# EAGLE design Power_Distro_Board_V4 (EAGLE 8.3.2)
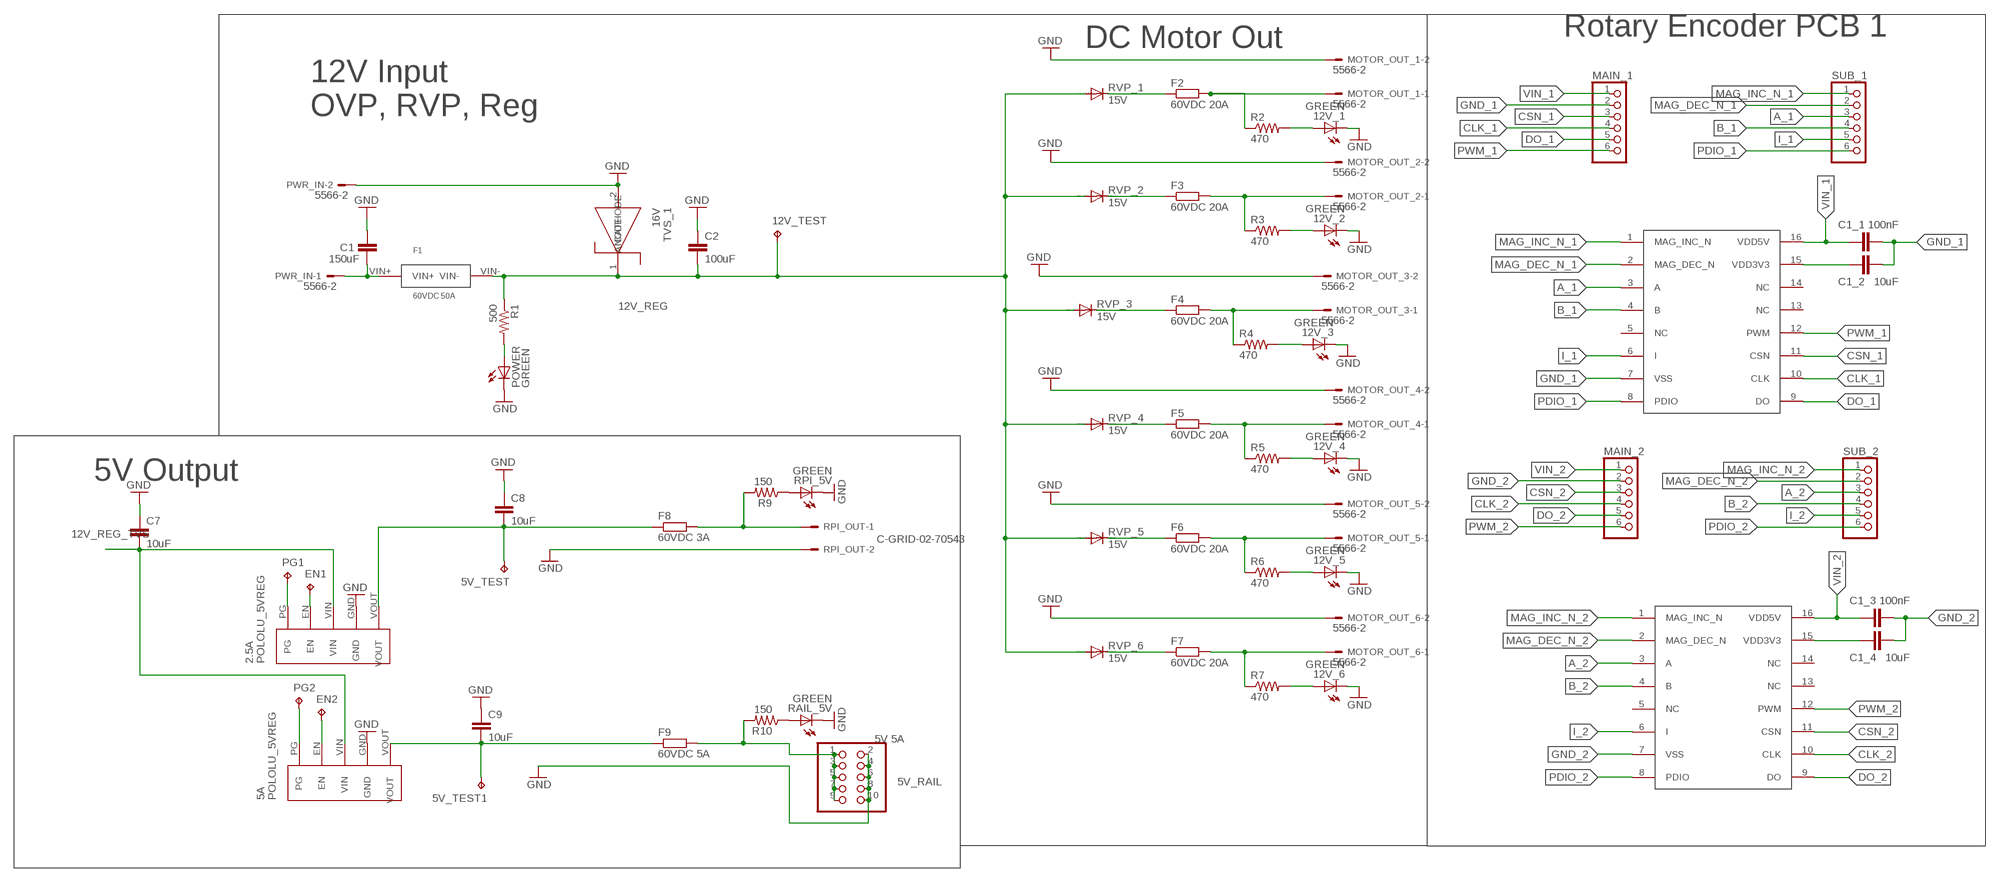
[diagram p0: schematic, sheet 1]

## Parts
2.5A  POLOLU_5VREG  [SIP5]
5A  POLOLU_5VREG  [SIP5]
5V_RAIL  5V 5A  PINHD-2X5  [2X05]
5V_TEST  TPPAD1-13  [P1-13]
5V_TEST1  TPPAD1-13  [P1-13]
12V_1  GREEN  LEDSML1206  [SML1206]
12V_2  GREEN  LEDSML1206  [SML1206]
12V_3  GREEN  LEDSML1206  [SML1206]
12V_4  GREEN  LEDSML1206  [SML1206]
12V_5  GREEN  LEDSML1206  [SML1206]
12V_6  GREEN  LEDSML1206  [SML1206]
12V_TEST  TPPAD1-13  [P1-13]
C1  150uF  C-EUC1206  [C1206]
C1_1  100nF  C-EUC1206  [C1206]
C1_2  10uF  C-EUC1206  [C1206]
C1_3  100nF  C-EUC1206  [C1206]
C1_4  10uF  C-EUC1206  [C1206]
C2  100uF  C-EUC1206  [C1206]
C7  10uF  C-EUC1206  [C1206]
C8  10uF  C-EUC1206  [C1206]
C9  10uF  C-EUC1206  [C1206]
EN1  TPPAD1-13  [P1-13]
EN2  TPPAD1-13  [P1-13]
ENC_1  ENCODER_AS5045B  [SSOP16]
ENC_2  ENCODER_AS5045B  [SSOP16]
F1  60VDC 50A  LITTLEFUSENANO463  [NANO]
F2  60VDC 20A  R-EU_R1206W  [R1206W]
F3  60VDC 20A  R-EU_R1206W  [R1206W]
F4  60VDC 20A  R-EU_R1206W  [R1206W]
F5  60VDC 20A  R-EU_R1206W  [R1206W]
F6  60VDC 20A  R-EU_R1206W  [R1206W]
F7  60VDC 20A  R-EU_R1206W  [R1206W]
F8  60VDC 3A  R-EU_R1206W  [R1206W]
F9  60VDC 5A  R-EU_R1206W  [R1206W]
MAIN_1  PINHD-1X6  [1X06]
MAIN_2  PINHD-1X6  [1X06]
MOTOR_OUT_1  5566-2  [5566-2]
MOTOR_OUT_2  5566-2  [5566-2]
MOTOR_OUT_3  5566-2  [5566-2]
MOTOR_OUT_4  5566-2  [5566-2]
MOTOR_OUT_5  5566-2  [5566-2]
MOTOR_OUT_6  5566-2  [5566-2]
PG1  TPPAD1-13  [P1-13]
PG2  TPPAD1-13  [P1-13]
POWER  GREEN  LEDSML1206  [SML1206]
PWR_IN  5566-2  [5566-2]
R1  500  R-US_R1206  [R1206]
R2  470  R-US_R1206  [R1206]
R3  470  R-US_R1206  [R1206]
R4  470  R-US_R1206  [R1206]
R5  470  R-US_R1206  [R1206]
R6  470  R-US_R1206  [R1206]
R7  470  R-US_R1206  [R1206]
R9  150  R-US_R1206  [R1206]
R10  150  R-US_R1206  [R1206]
RAIL_5V  GREEN  LEDSML1206  [SML1206]
RPI_5V  GREEN  LEDSML1206  [SML1206]
RPI_OUT  C-GRID-02-70543  [70543-02]
RVP_1  15V  BYT08P  [TO220ACS]
RVP_2  15V  BYT08P  [TO220ACS]
RVP_3  15V  BYT08P  [TO220ACS]
RVP_4  15V  BYT08P  [TO220ACS]
RVP_5  15V  BYT08P  [TO220ACS]
RVP_6  15V  BYT08P  [TO220ACS]
SUB_1  PINHD-1X6  [1X06]
SUB_2  PINHD-1X6  [1X06]
TVS_1  16V  SMAJ26A_TVSSMA  [DO-214AC]

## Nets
5V_REG: 2.5A.VOUT 5V_TEST.TP C8.2 F8.1
5V_REG1: F8.2 R9.2 RPI_OUT.1
5V_REG3: 5V_RAIL.1 5V_RAIL.3 5V_RAIL.5 5V_RAIL.7 5V_RAIL.9 F9.2 R10.2
12V_REG: 12V_TEST.TP C2.2 F1.VIN- R1.1 RVP_1.A RVP_2.A RVP_3.A RVP_4.A RVP_5.A RVP_6.A TVS_1.1(CATHODE)
12V_REG_TVS: 2.5A.VIN 5A.VIN C7.2
A_1: ENC_1.3(A) SUB_1.3
A_2: ENC_2.3(A) SUB_2.3
B_1: ENC_1.4(B) SUB_1.4
B_2: ENC_2.4(B) SUB_2.4
CLK_1: ENC_1.10(CLK) MAIN_1.4
CLK_2: ENC_2.10(CLK) MAIN_2.4
CSN_1: ENC_1.11(CSN) MAIN_1.3
CSN_2: ENC_2.11(CSN) MAIN_2.3
DO_1: ENC_1.9(DO) MAIN_1.5
DO_2: ENC_2.9(DO) MAIN_2.5
GND: 2.5A.GND 5A.GND 5V_RAIL.2 5V_RAIL.4 5V_RAIL.6 5V_RAIL.8 5V_RAIL.10 12V_1.C 12V_2.C 12V_3.C 12V_4.C 12V_5.C 12V_6.C C1.1 C2.1 C7.1 C8.1 C9.1 MOTOR_OUT_1.2 MOTOR_OUT_2.2 MOTOR_OUT_3.2 MOTOR_OUT_4.2 MOTOR_OUT_5.2 MOTOR_OUT_6.2 POWER.C PWR_IN.2 RAIL_5V.C RPI_5V.C RPI_OUT.2 TVS_1.2(ANODE)
GND_1: C1_1.2 C1_2.2 ENC_1.7(VSS) MAIN_1.2
GND_2: C1_3.2 C1_4.2 ENC_2.7(VSS) MAIN_2.2
I_1: ENC_1.6(I) SUB_1.5
I_2: ENC_2.6(I) SUB_2.5
MAG_DEC_N_1: ENC_1.2(MAG_DEC_N) SUB_1.2
MAG_DEC_N_2: ENC_2.2(MAG_DEC_N) SUB_2.2
MAG_INC_N_1: ENC_1.1(MAG_INC_N) SUB_1.1
MAG_INC_N_2: ENC_2.1(MAG_INC_N) SUB_2.1
N$1: POWER.A R1.2
N$2: 2.5A.PG PG1.TP
N$3: C1.2 F1.VIN+ PWR_IN.1
N$4: C1_2.1 ENC_1.15(VDD3V3)
N$5: F2.1 RVP_1.C
N$6: 2.5A.EN EN1.TP
N$7: F6.1 RVP_5.C
N$8: 5A.PG PG2.TP
N$9: 12V_1.A R2.2
N$10: R9.1 RPI_5V.A
N$11: R10.1 RAIL_5V.A
N$12: F2.2 MOTOR_OUT_1.1 R2.1
N$13: 12V_5.A R6.2
N$14: F3.1 RVP_2.C
N$15: 5A.EN EN2.TP
N$16: 12V_2.A R3.2
N$17: F6.2 MOTOR_OUT_5.1 R6.1
N$18: F3.2 MOTOR_OUT_2.1 R3.1
N$20: F7.1 RVP_6.C
N$21: 12V_6.A R7.2
N$22: F4.1 RVP_3.C
N$23: F7.2 MOTOR_OUT_6.1 R7.1
N$24: 12V_3.A R4.2
N$25: F4.2 MOTOR_OUT_3.1 R4.1
N$26: F5.1 RVP_4.C
N$27: 12V_4.A R5.2
N$28: F5.2 MOTOR_OUT_4.1 R5.1
N$29: C1_4.1 ENC_2.15(VDD3V3)
N$32: 5A.VOUT 5V_TEST1.TP C9.2 F9.1
PDIO_1: ENC_1.8(PDIO) SUB_1.6
PDIO_2: ENC_2.8(PDIO) SUB_2.6
PWM_1: ENC_1.12(PWM) MAIN_1.6
PWM_2: ENC_2.12(PWM) MAIN_2.6
VIN_1: C1_1.1 ENC_1.16(VDD5V) MAIN_1.1
VIN_2: C1_3.1 ENC_2.16(VDD5V) MAIN_2.1
Unconnected: ENC_1.5(NC) ENC_1.13(NC) ENC_1.14(NC) ENC_2.5(NC) ENC_2.13(NC) ENC_2.14(NC)

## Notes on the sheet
- **This encoder PCBs will be cut out of the main board
- Rotary Encoder PCB 1
- DC Motor Out
- 12V Input 
  OVP, RVP, Reg
- 5V Output
- **The ERC will say that there are no pins on net 12V_REG3, 
  which I have not been able to find anywhere. 
  
  It is not used anywhere too, 
  I think it's a bug in EAGLE.

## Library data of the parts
2.5A 5A = POWER_DISTRO:POLOLU_5VREG: Pololu 5V Regulator Variable Output Current
5V_RAIL = pinhead:PINHD-2X5: PIN HEADER
5V_TEST 5V_TEST1 12V_TEST EN1 EN2 PG1 PG2 = testpad:TP: Test pad
12V_1-12V_6 POWER RAIL_5V RPI_5V = led:LED: LED
C1 C1_1-C1_4 C2 C7-C9 = resistor:C-EU: CAPACITOR, European symbol
ENC_1 ENC_2 = minebot_PDR:ENCODER_AS5045B
F1 = minebot_PDR:LITTLEFUSENANO463
F2-F9 = resistor:R-EU_: RESISTOR, European symbol
MAIN_1 MAIN_2 SUB_1 SUB_2 = pinhead:PINHD-1X6: PIN HEADER
MOTOR_OUT_1-MOTOR_OUT_6 PWR_IN = con-molex:5566-2: Mini FIT connector 2 pol; OC_FARNELL: 1822072; OC_NEWARK: unknown
R1-R7 R9 R10 = resistor:R-US_: RESISTOR, American symbol
RPI_OUT = con-molex:C-GRID-02: CONNECTOR; OC_FARNELL: unknown; OC_NEWARK: unknown
RVP_1-RVP_6 = diode:BYT08P: DIODE
TVS_1 = POWER_DISTRO:SMAJ26A_TVS: TVS Diode, SMAJ26A

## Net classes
0 default: width 0.025 mm, drill 0.254 mm, clearance 0.254 mm
1 Power IN: width 4.801 mm
2 Motor_OUT: width 4.801 mm
3 3.3V_1A: width 0.305 mm
4 5V_1A: width 0.305 mm
5 12V_2A: width 0.813 mm

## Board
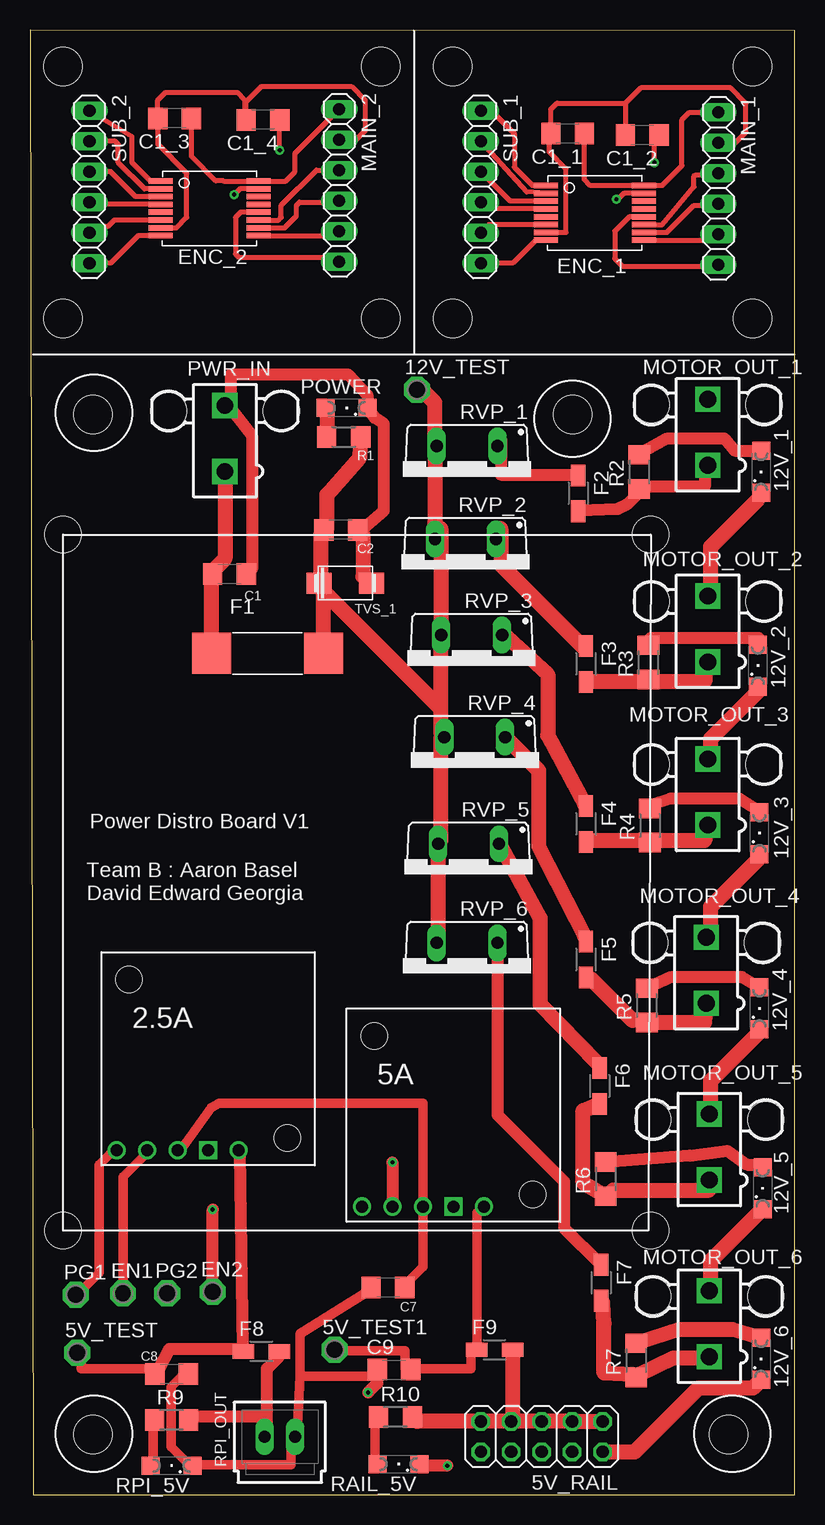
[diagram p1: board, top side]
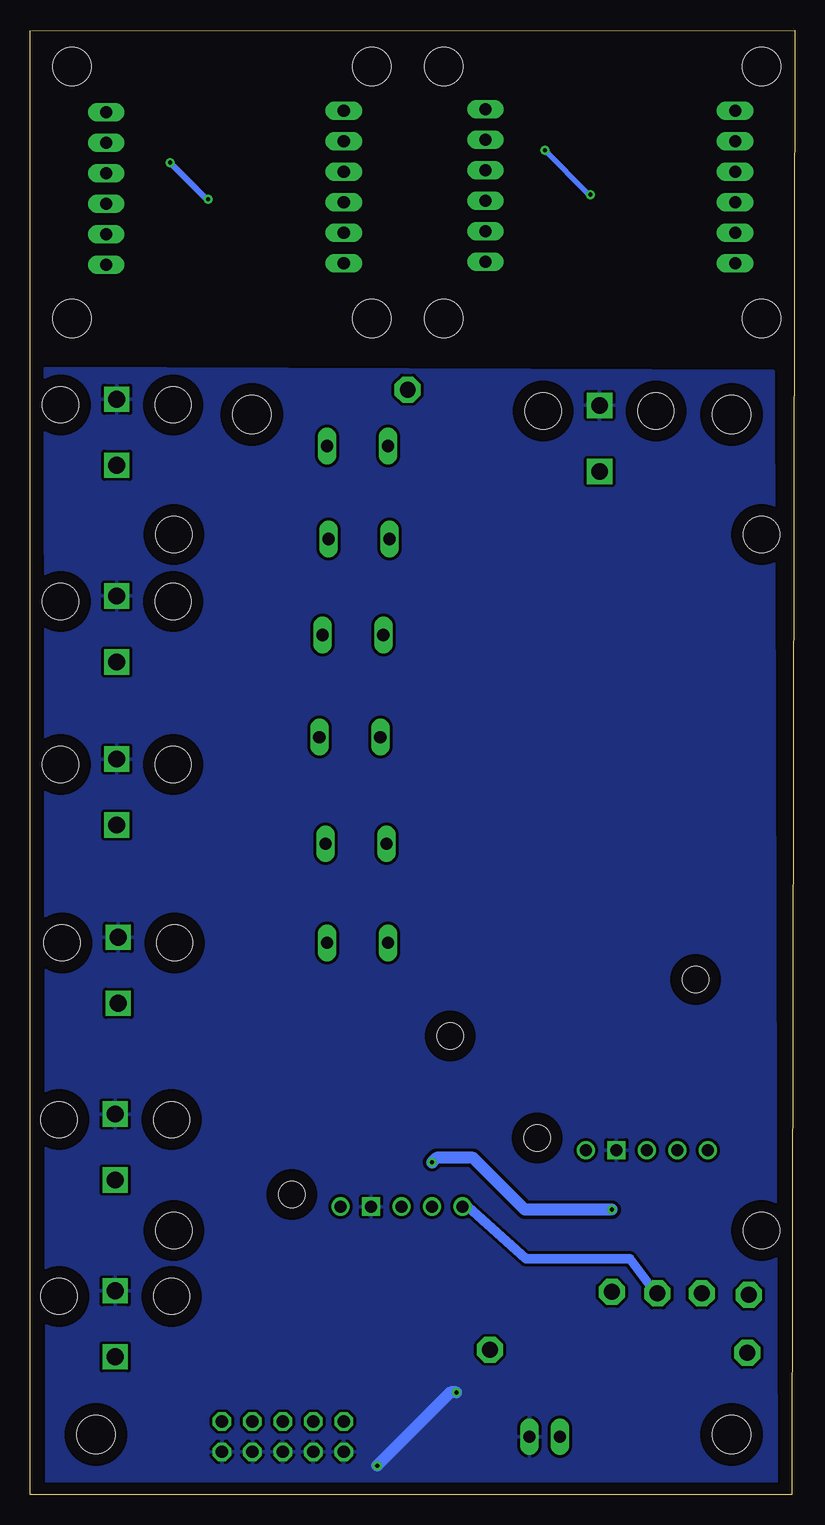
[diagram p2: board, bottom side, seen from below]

Size 63.75 x 122.05 mm. Coordinates in mm from the lower left corner, seen from the top.
Outline: 0.25,0 63.75,0 63.75,122 0,122.05 0.25,0
Copper layers (1*16): Top 0.035mm / dielectric 1.5mm / Bottom 0.035mm
Design rules "default *": minimum track width 6mil, minimum drill 0.35mm, track to track 6mil, track to pad 6mil, pad to pad 6mil, via to via 6mil, smd to smd 0mil, copper to edge 40mil, drill to drill 6mil, minimum pad ring 10mil, minimum via ring 8mil, stop-mask expansion 4mil, vias tented up to drill 0mil, thermal gap 10mil
Holes 3.17 mm at 5.25,5 58.25,5 45.25,90 5.25,90 35.25,98 60.25,98 60.25,119 35.25,119 2.75,98 29.25,98 29.25,119 2.75,119
Holes 3 mm at 2.75,80 51.75,80 51.75,22 2.75,22

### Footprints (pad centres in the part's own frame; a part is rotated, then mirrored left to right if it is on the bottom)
SIP5 = drill 1: EN -5.08,-7.62; PG -7.62,-7.62; VIN -2.54,-7.62; VOUT 2.54,-7.62 | drill 1 square: GND 0,-7.62 | hole 2.184: 6.604,-6.604; -6.604,6.604
2X05 = drill 1.016 octagon: 1 -5.08,-1.27; 2 -5.08,1.27; 3 -2.54,-1.27; 4 -2.54,1.27; 5 0,-1.27; 6 0,1.27; 7 2.54,-1.27; 8 2.54,1.27; 9 5.08,-1.27; 10 5.08,1.27
P1-13 = drill 1.321 pad 2.159 octagon: TP 0,0
SML1206 = smd 1.5 x 1.5: A 1.75,0; C -1.75,0
C1206 = smd 1.6 x 1.8: 1 -1.4,0; 2 1.4,0
SSOP16 = smd 2 x 0.46: 1 -4.08,2.275; 2 -4.08,1.625; 3 -4.08,0.975; 4 -4.08,0.325; 5 -4.08,-0.325; 6 -4.08,-0.975; 7 -4.08,-1.625; 8 -4.08,-2.275; 9 4.08,-2.275; 10 4.08,-1.625; 11 4.08,-0.975; 12 4.08,-0.325; 13 4.08,0.325; 14 4.08,0.975; 15 4.08,1.625; 16 4.08,2.275
NANO = smd 3.25 x 3.43: VIN+ -4.675,0; VIN- 4.675,0
R1206W = smd 1.8 x 1.2: 1 -1.499,0; 2 1.499,0
1X06 = drill 1.016 long: 1 -6.35,0; 2 -3.81,0; 3 -1.27,0; 4 1.27,0; 5 3.81,0; 6 6.35,0
5566-2 = drill 1.4 square: 1 0,-2.75; 2 0,2.75 | hole 3: 4.7,2.29; -4.7,2.29
R1206 = smd 1.6 x 1.803: 1 -1.422,0; 2 1.422,0
70543-02 = drill 1.016 long: 1 -1.27,0; 2 1.27,0
TO220ACS = drill 1.016 long: A 2.54,-2.54; C -2.54,-2.54
DO-214AC = smd 2.083 x 1.778: 1 -2.184,0; 2 2.184,0

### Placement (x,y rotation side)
2.5A  14.86,36.32 0 top
5A  35.31,31.62 0 top
5V_RAIL  42.67,4.83 180 top
5V_TEST  3.94,11.81 0 top
5V_TEST1  25.4,12.06 0 top
12V_1  60.96,85.22 90 top
12V_2  60.71,69.09 90 top
12V_3  60.83,55.12 90 top
12V_4  60.83,40.51 90 top
12V_5  61.09,25.53 90 top
12V_6  60.96,11.3 90 top
12V_TEST  32.26,92.08 0 top
C1  16.64,76.71 180 top
C1_1  44.83,113.41 180 top
C1_2  51.05,113.28 180 top
C1_3  12.06,114.68 180 top
C1_4  19.43,114.55 180 top
C2  25.91,80.39 180 top
C7  29.85,17.27 0 top
C8  11.81,10.03 180 top
C9  30.35,10.41 0 top
EN1  7.75,16.76 0 top
EN2  15.24,16.89 0 top
ENC_1  47.12,106.81 0 top
ENC_2  14.99,107.19 0 top
F1  19.81,70.1 0 top
F2  45.72,83.44 270 top
F3  46.35,69.22 270 top
F4  46.35,55.88 270 top
F5  46.35,44.58 270 top
F6  47.5,34.04 270 top
F7  47.62,17.65 270 top
F8  19.3,11.94 0 top
F9  38.73,12.06 0 top
MAIN_1  57.4,108.84 270 top
MAIN_2  25.78,109.09 270 top
MOTOR_OUT_1  56.52,88.52 0 top
MOTOR_OUT_2  56.52,72.14 0 top
MOTOR_OUT_3  56.52,58.55 0 top
MOTOR_OUT_4  56.39,43.69 0 top
MOTOR_OUT_5  56.64,28.96 0 top
MOTOR_OUT_6  56.64,14.22 0 top
PG1  3.81,16.64 0 top
PG2  11.43,16.76 0 top
POWER  26.42,90.55 180 top
PWR_IN  16.26,88.01 0 top
R1  26.16,88.14 180 top
R2  50.8,85.22 90 top
R3  51.56,69.34 90 top
R4  51.69,55.75 90 top
R5  51.43,40.77 90 top
R6  48.01,26.29 90 top
R7  50.55,11.18 90 top
R9  11.81,6.22 0 top
R10  30.48,6.48 0 top
RAIL_5V  30.73,2.54 180 top
RPI_5V  11.81,2.41 180 top
RPI_OUT  20.83,4.83 0 top
RVP_1  36.45,84.84 180 top
RVP_2  36.32,77.09 180 top
RVP_3  36.83,69.09 180 top
RVP_4  37.08,60.58 180 top
RVP_5  36.58,51.69 180 top
RVP_6  36.45,43.43 180 top
SUB_1  37.59,108.97 270 top
SUB_2  4.95,108.97 270 top
TVS_1  26.29,75.95 0 top

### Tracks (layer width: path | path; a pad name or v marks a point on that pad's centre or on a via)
5V_REG
  Top 0.8: 5V_TEST.TP 4.25,11.5 4.25,10.5 10.25,10.5 C8.2 10.75,10.5 | 17.5,28.5 2.5A.VOUT | 17.75,12.13 F8.1 17.75,12 17.75,12.13
  Top 1.016: 10.75,10.5 11.64,12.13 17.75,12.13 17.5,28.5
5V_REG1
  Top 0.8: 20.75,11.5 F8.2 | 19.75,5 RPI_OUT.1 | 13.25,6.5 R9.2
  Top 1.016: 20.75,11.5 19.75,10.5 19.75,6.5 | 19.75,5 19.75,6.5 | 19.75,6.5 13.25,6.5
5V_REG3
  Top 1.27: F9.2 40.23,6.2 5V_RAIL.7 | 5V_RAIL.7 42.8,6.1 5V_RAIL.3 5V_RAIL.1 | 5V_RAIL.5 5V_RAIL.7 | 5V_RAIL.7 5V_RAIL.9 32.28,6.1 R10.2
12V_REG
  Top 0.8: 24.25,80 C2.2 24.75,80.5 | 34.25,71.5 RVP_3.A 34.25,72 | 34.25,63.5 RVP_4.A 34.25,63 | 33.75,81 RVP_2.A 34.25,80.5 | 33.75,88 RVP_1.A 33.75,88.5 | 32.75,92 12V_TEST.TP | 24.25,75.5 TVS_1.1 24.25,76 24.49,75.77 | 34.25,54.5 RVP_5.A
  Top 1.27: 24.25,76 24.25,80 | 24.75,80.5 24.75,83.33 27.5,86.45 R1.1 | 34.25,63.5 34.25,65.5 | 34.25,65.5 34.25,71.5 | 33.75,88 33.75,81 | 32.75,92 33.75,91 33.75,88.5 | 34.25,80.5 34.25,72 | 34.25,65.5 24.25,75.5 | 34.25,54.5 34.25,63 | F1.VIN- 24.49,75.77 | RVP_5.A 34.04,46.1 RVP_6.A
12V_REG_TVS
  Top 0.8: C7.2 31.25,17.5 32.75,19 5A.VIN 32.75,24.5 32.75,32.63 15.75,32.63 15.12,32.25 12.75,29 2.5A.VIN
A_1
  Top 0.406: ENC_1.3 40.05,107.78 SUB_1.3
A_2
  Top 0.406: ENC_2.3 8.8,108.16 6.73,110.24 SUB_2.3
B_1
  Top 0.406: ENC_1.4 38.16,107.13 SUB_1.4
B_2
  Top 0.406: ENC_2.4 5.14,107.51 SUB_2.4
CLK_1
  Top 0.406: ENC_1.10 53.11,105.18 55.37,107.44 57.28,107.44
  Top 0.8: 57.28,107.44 MAIN_1.4
CLK_2
  Top 0.406: ENC_2.10 21.24,105.56 22.23,106.55 22.23,107.44 22.48,107.7 25.65,107.7 MAIN_2.4
CSN_1
  Top 0.406: ENC_1.11 52.75,105.83 55.37,108.97 55.37,109.86 55.5,109.98 57.28,109.98
  Top 0.8: 57.28,109.98 MAIN_1.3
CSN_2
  Top 0.406: ENC_2.11 20.74,106.21 20.96,106.43 20.96,107.44 23.88,110.36 MAIN_2.3
DO_1
  Top 0.406: ENC_1.9 56.91,104.53 MAIN_1.5
DO_2
  Top 0.406: ENC_2.9 25.41,104.91 MAIN_2.5
GND  (via drill 0.35)
  Top 0.8: 27.75,80.5 C2.1 27.75,80 | 27.75,76.5 28.25,76 TVS_1.2 | 60.75,23.5 12V_5.C | 56.75,17 MOTOR_OUT_6.2 | 60.75,38.5 12V_4.C | 56.75,32 MOTOR_OUT_5.2 | 60.75,53 12V_3.C | 56.75,46.5 MOTOR_OUT_4.2 | 60.75,67 12V_2.C | 56.75,61.5 MOTOR_OUT_3.2 | 60.75,83 12V_1.C | 56.75,75 MOTOR_OUT_2.2 | C8.1 12.75,10 11.75,9 11.75,4 13.25,2.5 RPI_5V.C 13.75,2.5 21.75,2.5 21.75,4.5 RPI_OUT.2 22.25,5 22.51,9.87 | 18.52,77.13 C1.1 | 16.75,90.5 PWR_IN.2 16.75,91 | 22.51,9.87 22.51,13.41 28.25,17 C7.1 | 22.51,9.87 28.75,9.87 C9.1
  Top 1.016: 27.75,80.5 29.51,82 29.51,89.21 28.75,89.71 POWER.C 28.13,91.61 26.51,93.36 16.75,93.36 16.75,91 | 18.52,77.13 18.52,88.23 16.75,90.5 | C9.1 28.95,9.27 v28.19,8.51 | v34.8,2.41 32.61,2.41 RAIL_5V.C
  Top 1.27: 27.75,80 27.75,76.5 | 60.75,23.5 56.75,19.5 56.75,17 | 60.75,38.5 56.75,34.5 56.75,32 | 60.75,53 56.75,49 56.75,46.5 | 60.75,67 56.75,63 56.75,61.5 | 60.75,83 56.75,79 56.75,75 | 5V_RAIL.2 50.42,3.56 55.75,8.89 60.3,8.89 12V_6.C
  Bottom 1.016: v28.19,8.51 28.7,8.51 v34.8,2.41
  pour Bottom: 1.78,93.6 1.52,0.64 62.36,0.89 62.48,93.85
GND_1
  Top 0.406: MAIN_1.2 58.8,112.65 59.69,113.54 59.69,115.95 58.42,117.22 50.93,117.22 49.66,115.95 | 49.66,115.95 C1_2.2 | C1_1.2 43.43,115.44 43.94,115.95 49.66,115.95 | ENC_1.7 44.68,105.18 44.7,105.16 44.7,110.49 43.31,111.89 43.31,113.29
  Top 0.8: C1_2.2 | 43.31,113.29 C1_1.2
GND_2
  Top 0.406: ENC_2.7 12.22,105.56 13.08,106.43 13.08,110.11 10.67,112.52 C1_3.2 10.66,116.2 11.3,116.84 17.27,116.84 17.91,116.2 17.91,114.68 C1_4.2 18.03,116.08 19.3,117.35 26.8,117.35 27.94,116.2 27.94,113.67 27.18,112.9 MAIN_2.2
I_1
  Top 0.406: ENC_1.6 38.27,105.83 SUB_1.5
I_2
  Top 0.406: ENC_2.6 7.03,106.21 6.48,105.66 5.46,105.66 SUB_2.5
MAG_DEC_N_1
  Top 0.406: ENC_1.2 41.43,108.56 SUB_1.2
MAG_DEC_N_2
  Top 0.406: ENC_2.2 9.55,108.81 7.37,111 7.37,112.52 7.11,112.78 SUB_2.2
MAG_INC_N_1
  Top 0.152: ENC_1.1 43.13,109.12 43,109.12
  Top 0.406: ENC_1.1 41.89,109.11 | SUB_1.1 38.48,115.32 40.39,113.41 40.39,110.62 41.88,109.12 43,109.12
MAG_INC_N_2
  Top 0.406: ENC_2.1 10.04,109.46 8.51,111 8.51,113.16 SUB_2.1
N$1
  Top 0.8: 24.75,90 24.63,90.48 POWER.A
  Top 1.27: 24.75,90 R1.2
N$2
  Top 0.8: 2.5A.PG 6.75,28.5 5.75,27.5 5.75,18.5 4.25,17 PG1.TP
N$3
  Top 0.8: 15.25,77 C1.2 15.14,76.61 | 16.25,85 PWR_IN.1
  Top 1.27: 15.25,77 16.25,78 16.25,85 | F1.VIN+ 15.14,76.61
N$4  (via drill 0.35)
  Top 0.406: ENC_1.15 49.5,108.43 49.02,107.95 v48.89,107.95 | v52.07,111 52.07,112.9
  Top 0.8: 52.07,112.9 C1_2.1
  Bottom 0.5: v48.89,107.95 49.02,107.95 v52.07,111
N$5
  Top 0.8: 45.25,85 F2.1 | 39.25,88 RVP_1.C
  Top 1.016: 45.25,85 39.25,85 39.25,88
N$6
  Top 0.8: 2.5A.EN 9.75,28.5 7.75,26.5 7.75,17 EN1.TP
N$7
  Top 0.8: 47.25,36 F6.1 | 39.25,54 RVP_5.C
  Top 1.27: 47.25,36 42.54,40.84 42.54,48.05 39.25,54
N$8
  Bottom 0.8: 5A.PG 27.25,24 22.38,19.64 13.75,19.64 11.75,17 PG2.TP
N$9
  Top 0.8: 60.75,87 12V_1.A | 51.25,87 R2.2
  Top 1.016: 60.75,87 58.76,87 57.88,88.01 53.16,88.01 51.25,87
N$10
  Top 0.8: RPI_5V.A 10.25,2.5 10.25,6 R9.1
N$11
  Top 0.8: RAIL_5V.A 28.75,3 28.75,6 R10.1
N$12
  Top 0.8: 45.75,82 F2.2 | 50.75,83.5 R2.1 51.25,84 | 56.25,85.5 MOTOR_OUT_1.1
  Top 1.016: 45.75,82 48.99,82.13 49.75,82.5 50.75,83.5 | 51.25,84 56.25,84 56.25,85.5
N$13
  Top 0.8: 60.75,27.5 12V_5.A
  Top 1.016: 60.75,27.5 59.78,27.5 58.13,28.64 54.98,28.25 R6.2
N$14
  Top 0.8: 46.25,70.5 F3.1 | 39.25,80.5 RVP_2.C
  Top 1.27: 46.25,70.5 39.25,77.5 39.25,80.5
N$15  (via drill 0.35)
  Top 1.016: EN2.TP v15.24,23.75 | v30.23,27.69 5A.EN
  Bottom 1.016: v15.24,23.75 22.48,23.75 26.8,28.07 29.85,28.07 v30.23,27.69
N$16
  Top 0.8: 60.75,71.38 12V_2.A | 51.75,71.38 R3.2
  Top 1.016: 51.75,71.38 60.75,71.38
N$17
  Top 0.8: 47.25,32.5 F6.2 | 47.75,25 R6.1 48.25,25 48.63,25.36
  Top 1.27: 47.25,32.5 46.12,32 46.12,26 47.75,25 | 48.63,25.36 56.63,25.36 MOTOR_OUT_5.1
N$18
  Top 0.8: 46.75,67.75 F3.2 | 51.25,67.75 R3.1 51.75,67.75
  Top 1.016: 56.25,69 MOTOR_OUT_2.1
  Top 1.27: 51.25,67.75 46.75,67.75 | 51.75,67.75 56.25,67.75 56.25,69
N$20
  Top 1.016: F7.1 44.53,22.25 44.53,26.1 38.99,31.64 RVP_6.C
N$21
  Top 1.27: 12V_6.A 58.59,13.76 54.18,13.76 R7.2
N$22
  Top 0.8: 46.25,57.5 F4.1 | 39.75,71.5 RVP_3.C
  Top 1.27: 46.25,57.5 43.17,63.25 43.17,68.34 39.75,71.5
N$23
  Top 0.8: 47.75,16 F7.2 | 50.25,10 R7.1 50.75,10
  Top 1.27: 47.75,16 47.86,14.25 47.86,10.11 50.25,10 | 50.75,10 53.67,11.38 56.76,11.38 MOTOR_OUT_6.1
N$24
  Top 0.8: 60.75,57 12V_3.A | 51.75,57.5 R4.2
  Top 1.016: 60.75,57 59.14,58.02 53.44,58.01 51.75,57.5
N$25
  Top 0.8: 46.75,54.5 F4.2 | 51.25,54.5 R4.1 51.75,54.5 | 56.25,55.5 MOTOR_OUT_3.1
  Top 1.27: 51.25,54.5 46.75,54.5 | 51.75,54.5 56.25,54.5 56.25,55.5
N$26
  Top 0.8: 46.25,46.5 F5.1 | 39.75,63 RVP_4.C
  Top 1.27: 46.25,46.5 42.41,54.03 42.41,60.35 39.75,63
N$27
  Top 1.016: 12V_4.A 59.36,43.13 53.53,43.13 R5.2
N$28
  Top 0.8: 50.25,39.5 51.25,39.5 R5.1 51.75,39.5 51.75,39.36 | 46.75,43 F5.2
  Top 1.27: 50.25,39.5 46.75,43 | 51.75,39.36 56.25,39.36 MOTOR_OUT_4.1
N$29  (via drill 0.35)
  Top 0.406: ENC_2.15 17.5,108.81 v17.02,108.33 | v20.83,112.01 C1_4.1
  Bottom 0.406: v17.02,108.33 17.14,108.33 v20.83,112.01
N$32
  Top 0.8: 5A.VOUT 37.75,24 37.25,23.5 37.25,12.5 F9.1 36.75,12 36.75,10.5 31.75,10.5 C9.2 31.25,10.5 31.25,12 25.75,12 5V_TEST1.TP
PDIO_1
  Top 0.406: ENC_1.8 42.17,104.53 40.26,102.62 SUB_1.6
PDIO_2
  Top 0.406: ENC_2.8 9.03,104.91 6.73,102.62 SUB_2.6
PWM_1
  Top 0.406: ENC_1.12 49.97,106.48 48.77,105.28 48.77,103 49.4,102.36 57.28,102.36
  Top 0.8: 57.28,102.36 MAIN_1.6
PWM_2
  Top 0.406: ENC_2.12 17.58,106.86 17.14,106.43 17.14,103.38 17.4,103.12 25.4,103.12 MAIN_2.6
VIN_1
  Top 0.406: MAIN_1.1 54.99,115.19 54.36,114.55 54.36,110.74 52.69,109.08 ENC_1.16 46.75,109.08 46.23,109.6 C1_1.1
  Top 0.8: C1_1.1
VIN_2
  Top 0.406: C1_3.1 13.46,111.51 15.49,109.47 16.13,109.47 16.14,109.46 ENC_2.16 21.33,109.46 22.1,110.24 22.1,111.76 MAIN_2.1

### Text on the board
tNames: Power Distro Board V1 | Team B : Aaron Basel / David Edward Georgia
